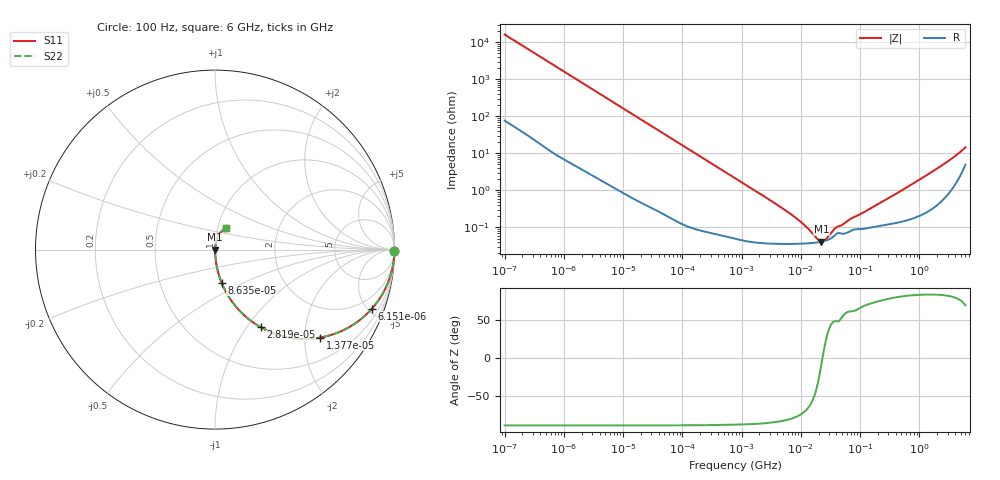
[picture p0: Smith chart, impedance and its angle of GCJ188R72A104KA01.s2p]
!Murata Part Number: GCJ188R72A104KA01
!These Parameters are Measured in Series Mode Connection
!Data Generated on Mar 13, 2026
!  o--ll--o
!Port1  Port2
!  o------o
!Operation Temp=25[degC], DC Bias Voltage=0[V]
!Freq. Start=100[Hz] Stop=6[GHz] 401[Steps]
# Hz S RI R 50
!Freq.(Hz) S11(Real) S11(Imag) S21(Real) S21(Imag) S12(Real) S12(Imag) S22(Real) S22(Imag)
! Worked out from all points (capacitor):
!   401 points, 100 Hz to 6 GHz, reference 50 ohm
!   read as one part in series: C = 98.3 nF near 109 Hz
!   lowest |Z| = 41.6 mohm at 22.26 MHz (marker M1)
!   series resonance near 23.23 MHz, so ESL is about 480 pH
!   S11 on the Smith chart (normalised r, x): 100 Hz: open; 6.151 kHz: 1.03, -5.32; 13.77 kHz: 1.01, -2.38; 28.19 kHz: 1.01, -1.17; 86.35 kHz: 1.00, -0.38; 6 GHz: 1.10, +0.27
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100  0.9999 -0.00619  6.75e-05 0.00619  6.75e-05 0.00619  0.9999 -0.00619
627  0.9984 -0.0385  0.00165 0.0385  0.00165 0.0385  0.9984 -0.0385
2008  0.9845 -0.1212  0.0155 0.1212  0.0155 0.1212  0.9845 -0.1212
6151  0.8748 -0.3284  0.1252 0.3284  0.1252 0.3284  0.8748 -0.3284
9204  0.7588 -0.4253  0.2412 0.4253  0.2412 0.4253  0.7588 -0.4253
13772  0.5859 -0.4899  0.4141 0.4899  0.4141 0.4899  0.5859 -0.4899
19704  0.4102 -0.489  0.5898 0.489  0.5898 0.489  0.4102 -0.489
28191  0.255 -0.4328  0.745 0.4328  0.745 0.4328  0.255 -0.4328
40335  0.1443 -0.3482  0.8557 0.3482  0.8557 0.3482  0.1443 -0.3482
86348  0.0365 -0.1839  0.9635 0.1839  0.9635 0.1839  0.0365 -0.1839
221108  0.00635 -0.0743  0.9937 0.0743  0.9937 0.0743  0.00635 -0.0743
774597  0.000954 -0.0215  0.999 0.0215  0.999 0.0215  0.000954 -0.0215
6353432  0.000364 -0.00244  0.9996 0.00244  0.9996 0.00244  0.000364 -0.00244
1.039699e7  0.000366 -0.00129  0.9996 0.00129  0.9996 0.00129  0.000366 -0.00129
1.555665e7  0.00038 -0.000594  0.9996 0.000594  0.9996 0.000594  0.00038 -0.000594
1.946e7  0.000396 -0.000257  0.9996 0.000257  0.9996 0.000257  0.000396 -0.000257
2.225763e7  0.000411 -6.17e-05  0.9996 6.17e-05  0.9996 6.17e-05  0.000411 -6.17e-05
2.662322e7  0.000442 0.000199  0.9996 -0.000199  0.9996 -0.000199  0.000442 0.000199
3.983537e7  0.000665 0.000759  0.9993 -0.000759  0.9993 -0.000759  0.000665 0.000759
3.124326e8  0.00125 0.0062  0.9987 -0.0062  0.9987 -0.0062  0.00125 0.0062
1.95892e9  0.00528 0.0376  0.9947 -0.0376  0.9947 -0.0376  0.00528 0.0376
6e9  0.0631 0.1218  0.9369 -0.1218  0.9369 -0.1218  0.0631 0.1218
